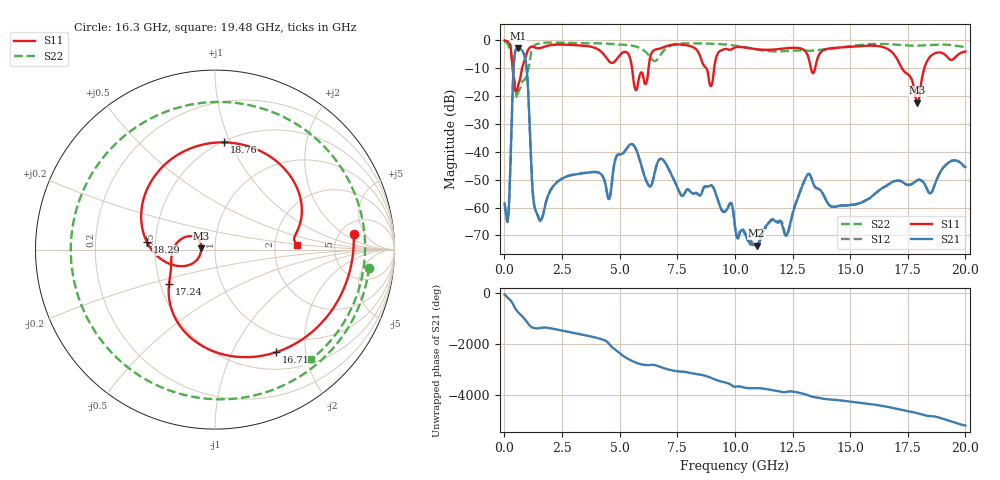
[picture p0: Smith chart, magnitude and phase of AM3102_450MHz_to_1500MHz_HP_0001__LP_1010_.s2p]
!Agilent Technologies,E8364B,MY43040894,A.07.50.67
!Agilent E8364B: A.07.50.67
!Date: Thursday, January 11, 2018 05:22:00
!Correction: S11(Full 2 Port(1,2))
!S21(Full 2 Port(1,2))
!S12(Full 2 Port(1,2))
!S22(Full 2 Port(1,2))
!S2P File: Measurements: S11, S21, S12, S22:
# Hz S  dB  R 50
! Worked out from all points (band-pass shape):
!   1601 points, 10 MHz to 20 GHz, reference 50 ohm
!   highest |S21| = -2.87 dB at 597.2 MHz (marker M1); lowest = -73.7 dB at 10.94 GHz (marker M2)
!   |S21| within 3 dB of the highest: 437.2 MHz to 882.9 MHz (445.6 MHz wide, 67.5 % of centre)
!   lowest |S11| = -22.4 dB at 17.91 GHz (marker M3), VSWR 1.16, Z = 42.9 + j0.578 ohm
!   |S11| at or under -10 dB: 356.9 MHz to 768.9 MHz (411.9 MHz wide, 73.2 % of centre); 5.538 GHz to 6.256 GHz (718.2 MHz wide, 12.2 % of centre); 17.25 GHz to 18.22 GHz (972.3 MHz wide, 5.48 % of centre)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
!   |S22| runs from -20.7 to -0.4 dB; largest |S21 - S12| = 0.0013
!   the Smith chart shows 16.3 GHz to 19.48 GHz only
!   S11 on the Smith chart (normalised r, x): 16.3 GHz: 6.63, +2.97; 16.71 GHz: 0.73, -1.51; 17.24 GHz: 0.56, -0.24; 18.29 GHz: 0.45, +0.05; 18.76 GHz: 0.51, +0.95; 19.48 GHz: 2.68, +0.19
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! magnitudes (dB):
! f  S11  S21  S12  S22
! 10 MHz  -0.1  -58.5  -59.0  -0.4
! 172.4 MHz  -0.6  -62.8  -62.8  -1.9
! 422.3 MHz  -15.1  -7.2  -7.2  -13.7
! 597.2 MHz  -16.1  -2.9  -2.9  -18.7
! 934.5 MHz  -5.5  -7.9  -7.9  -13.3
! 1.247 GHz  -2.3  -56.1  -56.1  -2.3
! 1.472 GHz  -2.9  -63.3  -63.5  -1.2
! 3.346 GHz  -1.9  -47.7  -47.7  -1.1
! 5.707 GHz  -17.9  -39.0  -39.0  -2.2
! 6.682 GHz  -3.1  -43.2  -43.2  -6.4
! 10.01 GHz  -2.5  -66.9  -67.1  -1.9
! 10.94 GHz  -3.2  -73.7  -73.8  -3.3
! 13.34 GHz  -11.3  -49.9  -50.0  -3.7
! 16.3 GHz  -2.2  -53.5  -53.5  -1.3
! 16.68 GHz  -3.3  -51.6  -51.6  -1.4
! 16.71 GHz  -3.5  -51.4  -51.4  -1.4
! 17.24 GHz  -9.9  -50.7  -50.6  -1.7
! 17.91 GHz  -22.4  -50.3  -50.2  -1.9
! 18.29 GHz  -8.4  -52.5  -52.6  -1.8
! 18.76 GHz  -4.4  -49.9  -49.9  -1.6
! 19.48 GHz  -6.8  -43.1  -43.1  -1.8
! 20 GHz  -4.0  -45.5  -45.6  -2.4
